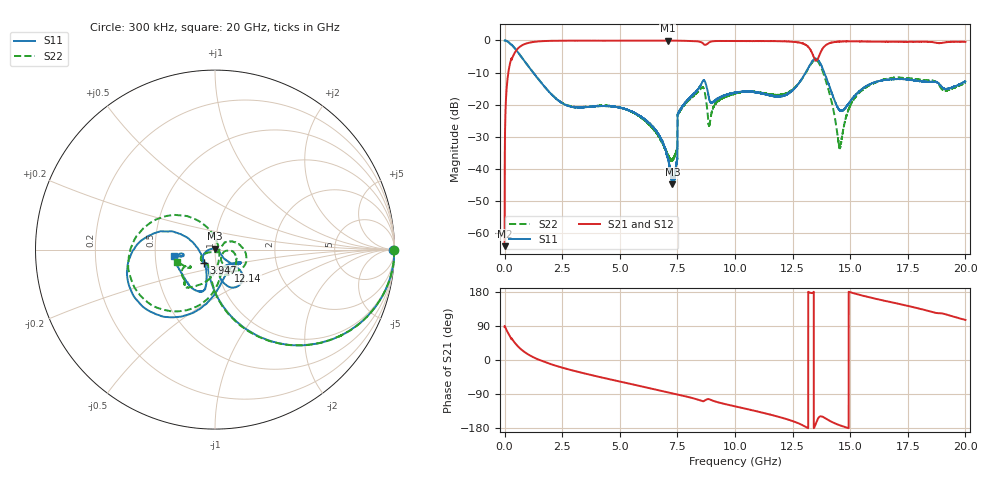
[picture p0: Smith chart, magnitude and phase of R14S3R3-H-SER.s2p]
!{R14S3R3}
!Johanson Technology Inc.
!www.johansontechnology.com
!Test Board Conditions:
!Substrate Type  RO4350B
!Substrate Thickness  20 mil
!Substrate Dk  3.66
!TL Type: GCPW
!TL Trace Width  36 mil
!TL Gap  12 mil
!Electrode orientation  Horizontal
!DUT TOPOLOGY	SERIES
!Mounting Pad LxW  26x36 mil
! Created Wed Nov 25 17:33:21 2020
! 2 Port Network Data from SP1.SP block
! freq  magS11  angS11  magS21  angS21  magS12  angS12  magS22  angS22
# khz S ma R 50
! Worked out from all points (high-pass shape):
!   20001 points, 300 kHz to 20 GHz, reference 50 ohm
!   highest |S21| = -0.04 dB at 7.084 GHz (marker M1); lowest = -63.9 dB at 300 kHz (marker M2)
!   |S21| within 3 dB of the highest: 511.2 MHz to 13.28 GHz (12.77 GHz wide, 185 % of centre); 13.76 GHz to end of sweep
!   lowest |S11| = -44.7 dB at 7.287 GHz (marker M3), VSWR 1.01, Z = 49.9 + j0.56 ohm
!   |S11| at or under -10 dB: 1.242 GHz to 13.07 GHz (11.83 GHz wide, 165 % of centre); 13.88 GHz to end of sweep
!   |S22| runs from -37.5 to 0.0 dB; largest |S21 - S12| = 0.018
!   S11 on the Smith chart (normalised r, x): 300 kHz: open; 3.947 GHz: 0.88, -0.13; 12.14 GHz: 1.12, -0.27; 20 GHz: 0.63, -0.05
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300  0.9925 -0.3  0.0006354 87.0  0.00061 88.1  0.9982 -0.2
125300  0.9673 -15.7  0.2509 74.1  0.2518 74.2  0.9669 -15.7
432300  0.7648 -43.4  0.6392 46.3  0.6403 46.2  0.7649 -43.5
1320300  0.291 -84.5  0.9546 5.2  0.9542 5.1  0.2922 -84.9
3334300  0.09116 -123.5  0.993 -33.4  0.9934 -33.4  0.09245 -121.5
3947300  0.09488 -130.1  0.9913 -42.4  0.9924 -42.4  0.09602 -132.9
6667300  0.03494 -176.9  0.9936 -79.3  0.9937 -79.3  0.03268 -152.5
7084300  0.01486 160.2  0.9955 -85.1  0.9934 -85.0  0.0167 -126.4
7287300  0.005788 103.9  0.9935 -87.9  0.9934 -87.9  0.01375 -85.2
7399300  0.00865 44.1  0.9936 -89.5  0.9934 -89.4  0.0165 -62.4
7600300  0.08149 -43.1  0.9894 -92.3  0.9895 -92.2  0.07901 33.1
7758300  0.09775 -42.1  0.9888 -94.5  0.9875 -94.5  0.09574 28.5
8584300  0.2267 -47.0  0.9166 -108.6  0.9159 -108.6  0.1868 -22.5
8906300  0.1132 -70.2  0.9446 -104.1  0.9446 -104.1  0.05095 -14.5
1.00003e7  0.1547 -26.7  0.9796 -122.3  0.9792 -122.3  0.1492 -41.8
1.21413e7  0.1394 -58.6  0.9689 -154.3  0.9709 -154.2  0.1472 -78.0
1.33343e7  0.4664 -126.5  0.6517 176.7  0.6539 176.4  0.4478 -132.4
1.38093e7  0.3631 166.6  0.7536 -149.8  0.7487 -150.3  0.3282 145.2
1.45523e7  0.08131 -164.7  0.9614 -172.4  0.9627 -172.3  0.02192 6.3
1.52453e7  0.1441 -109.2  0.9658 174.6  0.9694 174.5  0.134 -93.0
1.66673e7  0.2449 -108.8  0.9591 154.0  0.9513 153.8  0.2584 -124.7
2e7  0.2318 -170.8  0.9502 105.7  0.9496 105.9  0.2208 -162.3
